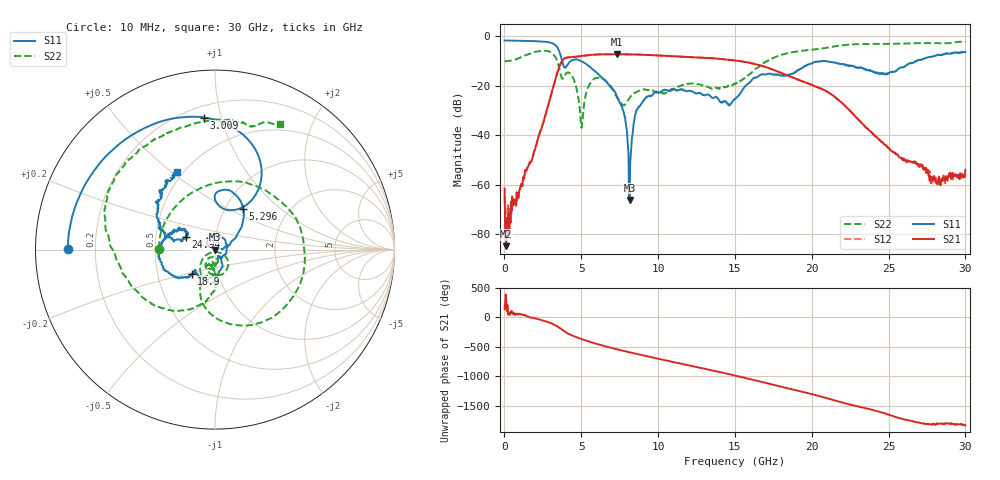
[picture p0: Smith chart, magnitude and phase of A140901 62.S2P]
!  2-Port S-parameters saved by WinCal
! VAR MeasName=S-Parameters (CALIBRATED_DATA) read from VNA (N5244A)
! VAR MeasDate=11/3/2014 9:36:48 AM
! VAR NAME=A140901 62
! VAR FILENAME=A140901 62.S2P
! VAR DATE=11/3/2014 9:36:48 AM
! VAR PHYS_PORTS=1,2
# Hz S RI R 50
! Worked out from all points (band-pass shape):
!   801 points, 10 MHz to 30 GHz, reference 50 ohm
!   highest |S21| = -7.27 dB at 7.32 GHz (marker M1); lowest = -84.8 dB at 122.5 MHz (marker M2)
!   |S21| within 3 dB of the highest: 3.721 GHz to 15.53 GHz (11.81 GHz wide, 123 % of centre)
!   lowest |S11| = -66.1 dB at 8.145 GHz (marker M3), VSWR 1.00, Z = 50 - j0.036 ohm
!   |S11| at or under -10 dB: 3.753 GHz to 4.321 GHz (567.6 MHz wide, 14.1 % of centre); 4.972 GHz to 20.66 GHz (15.68 GHz wide, 122 % of centre); 20.87 GHz to 26.83 GHz (5.955 GHz wide, 25 % of centre)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
!   |S22| runs from -36.9 to -2.1 dB; largest |S21 - S12| = 0.0017
!   S11 on the Smith chart (normalised r, x): 10 MHz: 0.10, +0.00; 3.009 GHz: 0.27, +0.88; 5.296 GHz: 1.21, +0.60; 18.9 GHz: 0.75, -0.21; 24.94 GHz: 0.71, +0.11; 30 GHz: 0.47, +0.52
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1e7  -0.8196 0.0018  -0.000618 0.000572  -0.000374 0.000422  -0.3121 0.00609
1.224625e8  -0.8186 0.0398  -1.18e-05 -5.66e-05  0.0001 -3.86e-05  -0.3078 0.0653
1.434525e9  -0.6694 0.4449  0.00179 0.000759  0.0018 0.000768  0.2117 0.358
3.009e9  -0.0598 0.7359  -0.0063 -0.0614  -0.00645 -0.0613  0.2353 -0.4124
4.133625e9  0.0019 0.2732  0.0206 0.3721  0.0202 0.3721  -0.0196 -0.1843
5.033325e9  0.1377 0.2776  0.3934 -0.0671  0.3934 -0.0668  0.00373 -0.0137
5.295738e9  0.1571 0.2286  0.3435 -0.2215  0.3437 -0.2212  0.0563 -0.0355
6.120462e9  0.1349 0.1032  -0.0654 -0.4231  -0.0649 -0.4226  0.0156 -0.1427
7.320062e9  0.0592 0.0166  -0.4327 0.0142  -0.4324 0.0135  -0.0354 -0.0468
7.8074e9  0.0247 0.00296  -0.3614 0.2331  -0.3611 0.2325  9.03e-05 -0.0411
8.144788e9  -0.000339 -0.00036  -0.2549 0.345  -0.2548 0.3447  0.0139 -0.0545
8.632125e9  -0.0304 0.0136  -0.0504 0.4235  -0.0505 0.4231  0.0113 -0.0754
1.001916e10  -0.0381 0.0632  0.3927 0.115  0.3918 0.1148  -0.0129 -0.0727
1.2006e10  0.0496 0.0611  -0.0303 -0.3794  -0.0307 -0.3786  -0.0223 -0.1079
1.346801e10  0.0505 -0.0294  -0.3597 -0.016  -0.3593 -0.0167  -0.0331 -0.0816
1.5005e10  0.0279 -0.0455  -0.0108 0.323  -0.0103 0.3227  -0.00783 -0.1102
1.89037e10  -0.1295 -0.1342  -0.1259 -0.062  -0.1258 -0.0629  -0.4073 -0.263
2.002832e10  -0.2545 -0.1308  -0.071 0.0745  -0.0719 0.0741  -0.5222 -0.1088
2.493919e10  -0.1636 0.0715  -0.00504 0.00288  -0.00493 0.00284  -0.2793 0.6445
2.501416e10  -0.1636 0.0639  -0.00456 0.00318  -0.00436 0.00317  -0.2663 0.6504
2.82006e10  -0.3308 0.2642  0.00118 -8.36e-05  0.000999 -0.000168  0.1602 0.7059
3e10  -0.2092 0.4316  0.00158 -0.00125  0.00137 -0.000749  0.3616 0.6995
